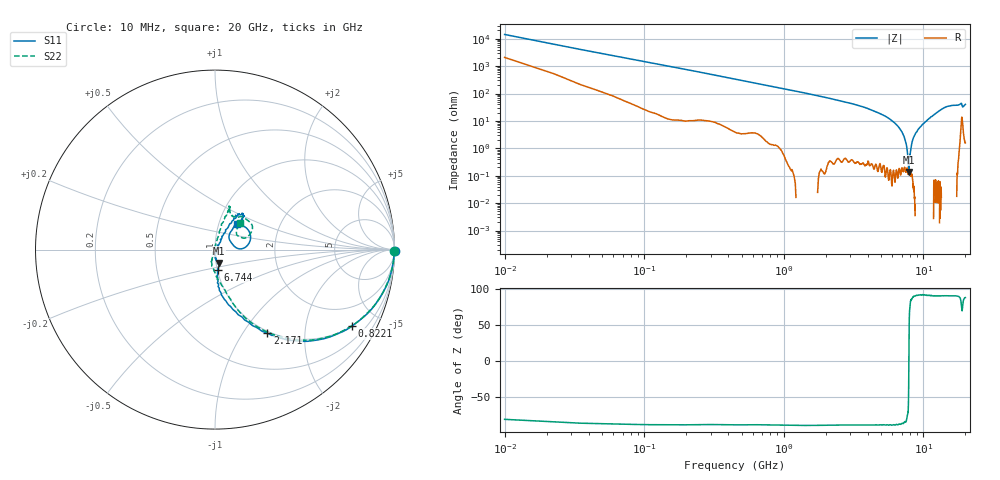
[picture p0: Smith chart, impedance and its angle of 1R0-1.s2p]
!Keysight Technologies,P5008B,MY61100088,A.16.20.02
!Date: Monday, May 27, 2024 13:42:52
!Correction: S11(C  2-Port  )
!S21(C  2-Port  )
!S12(C  2-Port  )
!S22(C  2-Port  )
!S2P File: Measurements: S11, S21, S12, S22:
# Hz S  dB  R 50
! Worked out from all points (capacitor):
!   1601 points, 10 MHz to 20 GHz, reference 50 ohm
!   read as one part in series: C = 1.06 pF near 110 MHz
!   lowest |Z| = 138 mohm at 7.856 GHz (marker M1)
!   series resonance near 7.869 GHz, so ESL is about 380 pH
!   S11 on the Smith chart (normalised r, x): 10 MHz: open; 822.1 MHz: 0.99, -3.60; 2.171 GHz: 0.97, -1.30; 6.744 GHz: 1.01, -0.23; 20 GHz: 1.23, +0.36
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1e7  0.01 -0.4  -43.08 81.2  -43.04 81.2  -0.02 -0.4
1.349375e8  -0.06 -5.3  -20.88 84.0  -20.89 84.0  -0.05 -5.3
2.473812e8  -0.14 -9.6  -15.83 79.5  -15.84 79.5  -0.14 -9.4
4.722688e8  -0.45 -17.7  -10.53 71.7  -10.54 71.8  -0.44 -17.5
8.220938e8  -1.16 -29.1  -6.45 60.7  -6.46 60.7  -1.14 -28.6
2.171419e9  -5.19 -57.9  -1.56 32.1  -1.57 32.1  -5.13 -56.8
3.345831e9  -8.54 -71.0  -0.64 19.3  -0.65 19.3  -8.62 -68.6
6.681662e9  -18.76 -81.7  -0.03 -0.0  -0.05 -0.0  -18.75 -92.9
6.744131e9  -19.01 -81.8  -0.03 -0.2  -0.04 -0.3  -19.00 -92.9
7.856075e9  -22.22 -74.9  0.00 -4.1  -0.00 -4.1  -22.70 -105.5
1.0005e10  -29.70 -88.3  0.04 -10.9  0.03 -10.9  -30.07 -107.9
1.050475e10  -34.14 -78.3  0.05 -12.3  0.04 -12.4  -33.89 -122.1
1.075462e10  -39.77 -24.2  0.05 -13.1  0.04 -13.1  -40.45 -161.8
1.095452e10  -38.08 26.3  0.05 -13.7  0.04 -13.7  -45.36 122.4
1.134183e10  -30.72 59.4  0.05 -14.9  0.04 -14.9  -32.63 81.1
1.194153e10  -24.02 59.8  0.03 -16.6  0.02 -16.6  -24.92 77.3
1.334083e10  -16.35 59.6  -0.04 -20.7  -0.05 -20.7  -16.44 74.7
1.477761e10  -12.58 57.5  -0.17 -24.9  -0.18 -24.9  -12.58 70.5
1.667666e10  -12.46 49.6  -0.18 -29.1  -0.19 -29.1  -12.43 70.2
1.866317e10  -13.41 22.5  -0.85 -36.8  -0.86 -36.7  -12.28 43.0
1.917541e10  -20.22 30.1  -0.57 -30.8  -0.58 -30.9  -16.18 27.7
2e10  -14.43 48.8  -0.24 -36.2  -0.25 -36.2  -13.88 46.4
